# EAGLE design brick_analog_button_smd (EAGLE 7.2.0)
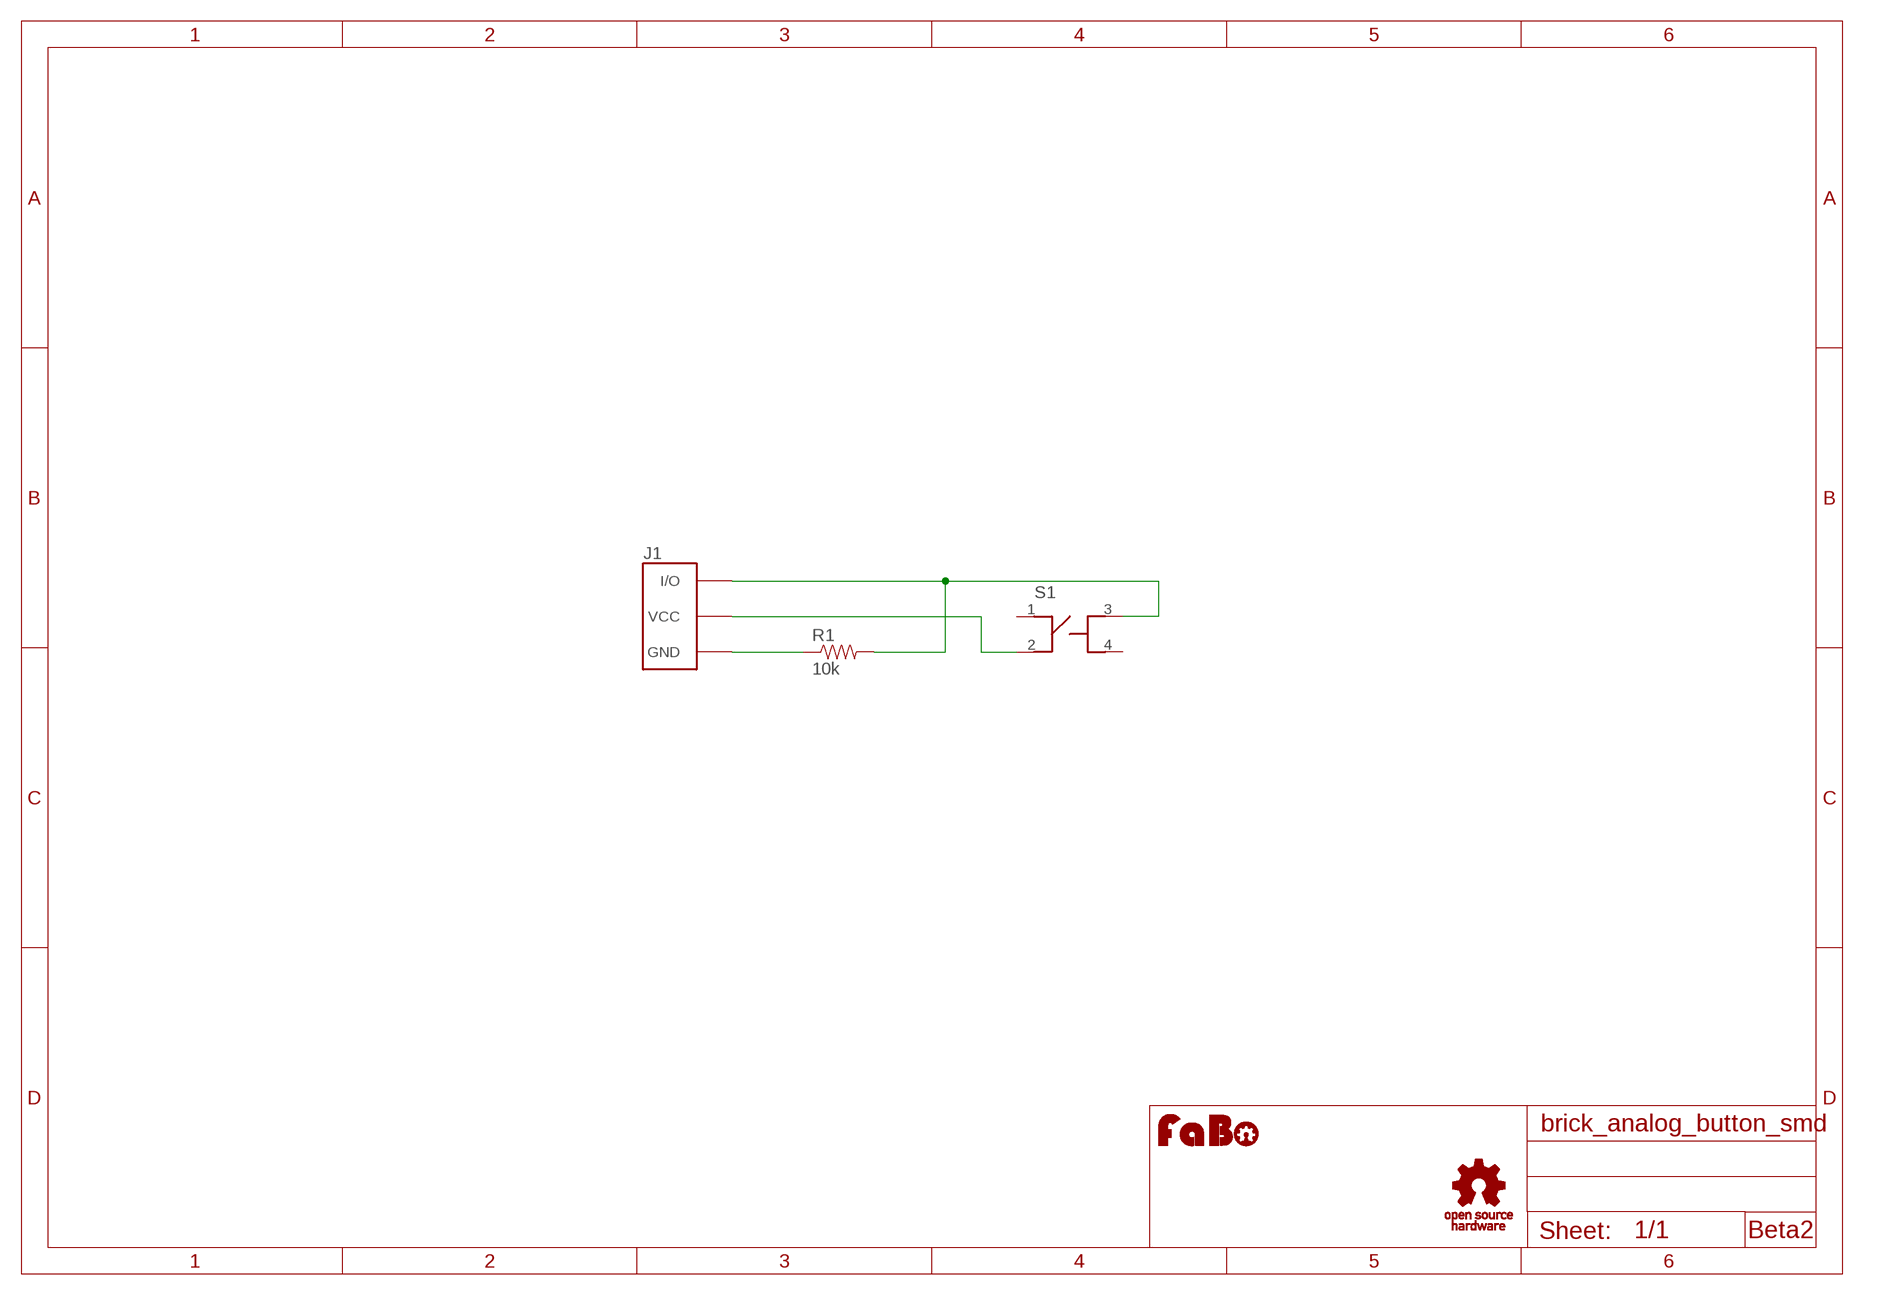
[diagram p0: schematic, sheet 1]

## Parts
J1  BRICK_3PIN  [BRICK_3PIN]
R1  10k  RESISTOR0603  [0603-RES]
S1  SWITCH-LS6J2M-T  [SWITCH-LS6J2M-T]
U$1  LOGO_FABO-M  [LOGO_FABO_M]
U$4  LOGO_OSHW_T-M  [LOGO_OSHW_T_M]

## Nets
GND: J1.GND R1.1
N$1: J1.VCC S1.2
N$3: J1.IN/OUT(I/O) R1.2 S1.3
Unconnected: S1.1 S1.4

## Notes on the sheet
- Beta2

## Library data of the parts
J1 = gclue:BRICK_3PIN: FaBo Brick 3pin
R1 = SparkFun-Resistors:RESISTOR: Resistor
S1 = gclue:SWITCH-LS6J2M-T: Switch Tact SMD(LS6J2M-T)
U$1 = FaBo:LOGO_FABO
U$4 = gclue:LOGO_OSHW_T

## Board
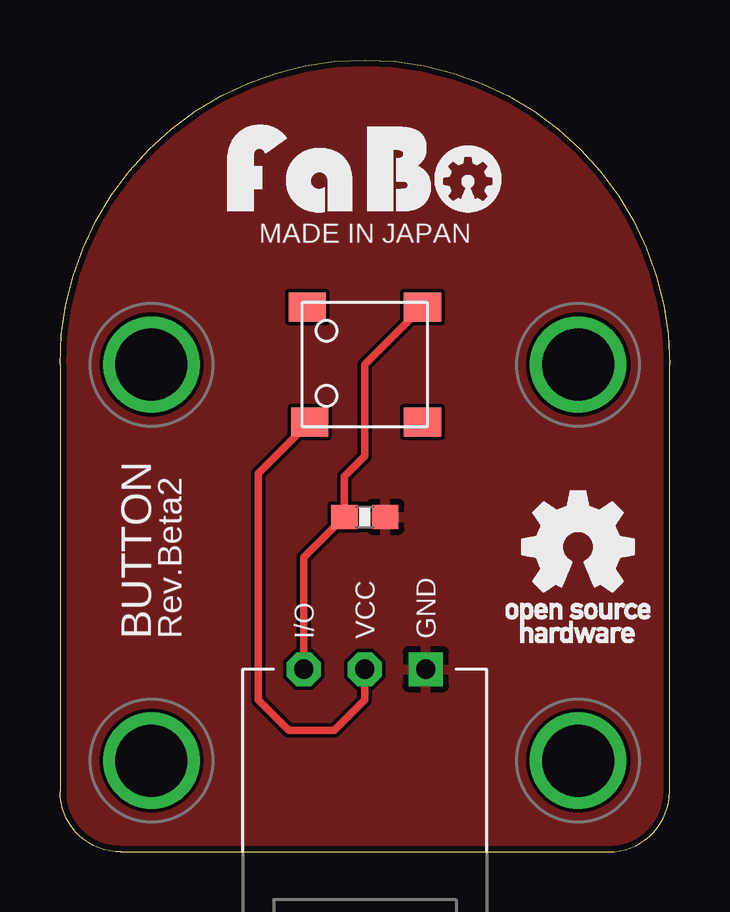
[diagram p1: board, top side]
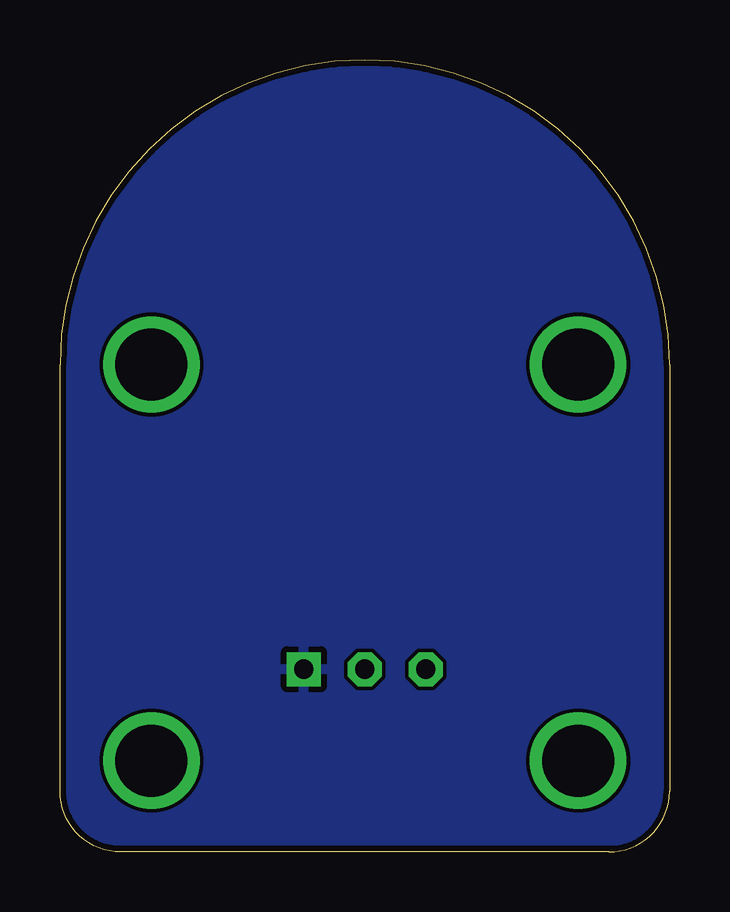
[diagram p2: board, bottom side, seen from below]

Size 25.4 x 33.02 mm. Coordinates in mm from the lower left corner, seen from the top.
Copper layers (1*16): Top 0.035mm / dielectric 1.5mm / Bottom 0.035mm
Design rules "Elecrow_2-layer_eagle_rule": minimum track width 6mil, minimum drill 12mil, track to track 6mil, track to pad 6mil, pad to pad 6mil, via to via 6mil, smd to smd 0mil, copper to edge 10mil, drill to drill 10mil, minimum pad ring 10mil, minimum via ring 6mil, stop-mask expansion 2mil, vias tented up to drill 100mil, thermal gap 10mil

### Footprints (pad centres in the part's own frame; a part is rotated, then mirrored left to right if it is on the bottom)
BRICK_3PIN = drill 0.8 pad 1.422 square: GND 2.54,-8.89 | drill 0.8 pad 1.422 octagon: IN/OUT -2.54,-8.89; VCC 0,-8.89 | drill 3 pad 3.81: P$5 -8.89,3.81; P$6 8.89,3.81; P$7 -8.89,-12.7; P$8 8.89,-12.7
0603-RES = smd 1.1 x 1: 1 -0.85,0; 2 0.85,0
SWITCH-LS6J2M-T = smd 1.55 x 1.2: 1 -2.4,2.4; 2 -2.3,-2.4; 3 2.4,2.4; 4 2.4,-2.4

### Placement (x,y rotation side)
J1  12.7,16.51 0 top
R1  12.7,13.97 180 top
S1  12.7,20.32 0 top
U$1  12.7,26.67 0 top
U$4  21.59,12.7 0 top

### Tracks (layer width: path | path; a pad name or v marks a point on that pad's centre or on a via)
GND
  pour Bottom: -1.27,-1.27 26.67,-1.27 26.67,34.29 -1.27,34.29
  pour Top: -1.27,-1.27 26.67,-1.27 26.67,34.29 -1.27,34.29
N$1
  Top 0.305: S1.2 8.26,15.78 8.26,6.35 9.53,5.08 11.43,5.08 12.7,6.35 J1.VCC
N$3
  Top 0.305: J1.IN/OUT 10.16,12.28 R1.2 11.85,15.66 12.7,16.51 12.7,20.32 S1.3

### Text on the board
tPlace: MADE IN JAPAN | BUTTON | Rev.Beta2

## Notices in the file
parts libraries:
SparkFun-Resistors: Licensing: Creative Commons ShareAlike 4.0 International - https://creativecommons.org/licenses/by-sa/4.0
